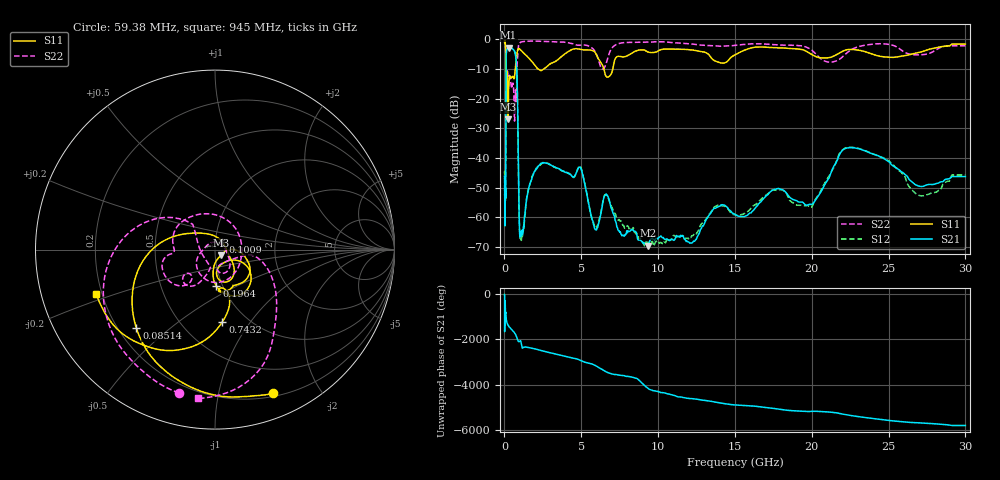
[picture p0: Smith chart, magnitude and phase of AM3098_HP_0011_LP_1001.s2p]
! Date/Time: Thu, Feb 28, 2019 8:34 AM
! Network Analyzer: Agilent Technologies E8364B Rev: A.07.50.67
! Sweep from 0.010 to 30.000 GHz, 1601 Points, Sweep Type: LOG
! Power Supply: 5.022 V, 0.002 A
# Hz S DB R 50
!freq MagS11 AngS11 MagS21 AngS21 MagS12 AngS12 MagS22 AngS22
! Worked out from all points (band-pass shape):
!   1601 points, 10 MHz to 30 GHz, reference 50 ohm
!   highest |S21| = -2.78 dB at 266.5 MHz (marker M1); lowest = -69.6 dB at 9.349 GHz (marker M2)
!   |S21| within 3 dB of the highest: 108.6 MHz to 735.3 MHz (626.6 MHz wide, 149 % of centre)
!   lowest |S11| = -26.9 dB at 233.9 MHz (marker M3), VSWR 1.09, Z = 53.2 - j3.4 ohm
!   |S11| at or under -10 dB: 93.02 MHz to 701.6 MHz (608.6 MHz wide, 153 % of centre); 2.192 GHz to 2.55 GHz (357.7 MHz wide, 15.1 % of centre); 6.473 GHz to 7.046 GHz (573.1 MHz wide, 8.48 % of centre)
!   |S22| runs from -27.5 to -0.5 dB; largest |S21 - S12| = 0.01
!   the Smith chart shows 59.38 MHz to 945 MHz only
!   S11 on the Smith chart (normalised r, x): 59.38 MHz: 0.23, -1.46; 85.14 MHz: 0.27, -0.39; 100.9 MHz: 1.08, +0.09; 196.4 MHz: 0.93, -0.40; 743.2 MHz: 0.78, -0.74; 945 MHz: 0.18, -0.17
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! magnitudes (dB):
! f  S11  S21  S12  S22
! 10 MHz  -0.3  -46.1  -45.2  -0.6
! 38.04 MHz  -0.5  -61.4  -61.8  -1.0
! 59.38 MHz  -1.3  -52.1  -52.9  -1.7
! 74.38 MHz  -2.1  -52.8  -51.5  -2.6
! 85.14 MHz  -4.2  -32.6  -32.2  -4.6
! 100.9 MHz  -24.5  -8.1  -8.1  -21.8
! 144.7 MHz  -15.5  -3.5  -3.5  -13.1
! 196.4 MHz  -13.8  -3.1  -3.1  -10.6
! 233.9 MHz  -26.9  -2.9  -2.8  -12.5
! 266.5 MHz  -17.6  -2.8  -2.7  -12.9
! 550.5 MHz  -12.5  -3.3  -3.3  -14.7
! 743.2 MHz  -7.9  -6.1  -6.1  -20.7
! 833.9 MHz  -4.2  -15.9  -15.9  -7.6
! 945 MHz  -3.0  -56.8  -56.9  -1.6
! 1.132 GHz  -3.9  -65.9  -66.3  -0.8
! 2.084 GHz  -9.4  -43.6  -43.3  -0.6
! 4.903 GHz  -3.3  -43.0  -42.7  -2.0
! 7.926 GHz  -5.7  -65.4  -63.0  -1.0
! 9.349 GHz  -4.2  -69.6  -68.4  -0.9
! 19.61 GHz  -3.9  -55.9  -56.2  -2.5
! 22.67 GHz  -3.4  -36.5  -36.4  -3.2
! 30 GHz  -1.6  -46.3  -45.7  -2.1
